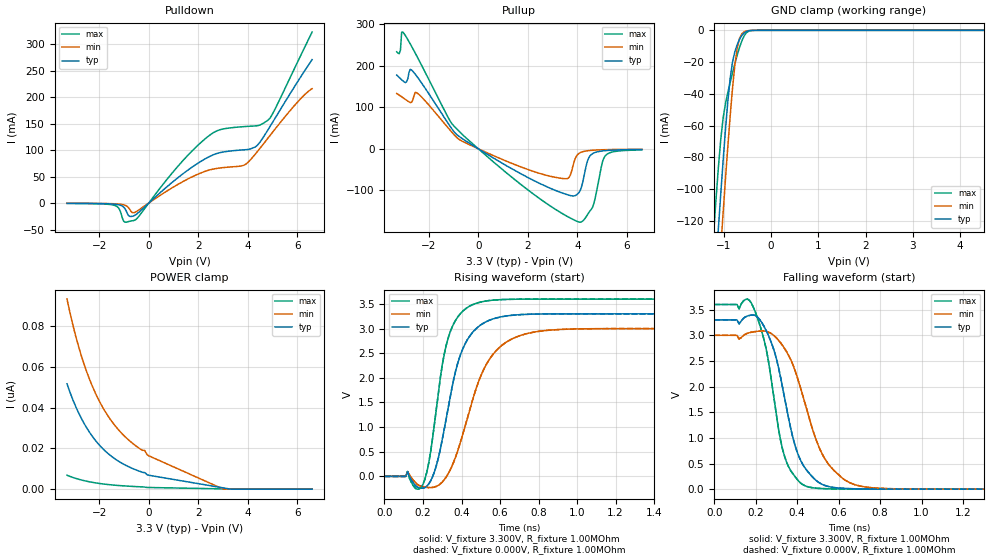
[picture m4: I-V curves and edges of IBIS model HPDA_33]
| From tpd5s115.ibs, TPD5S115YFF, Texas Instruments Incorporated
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[Model]   HPDA_33
Model_type   I/O
Vinl = 0.4V
Vinh = 1.0V
Vmeas = 1.500V
Vref = 0V
Cref =15pF
|   typ   min   max
|3-state
C_comp   1.7706pF   1.6054pF   2.0294pF
|pulldown
|C_comp   1.8194pF   1.5857pF   2.1620pF
|pullup
|C_comp   1.7863pF   1.5802pF   2.1259pF
[Voltage Range]   3.300V   3.000V   3.600V
|Junction temperature
[Temperature Range]   40.0   100.0   -40.0
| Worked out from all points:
|   slope of the pulldown table from 0 to 0.495 V, typ, clamps not added: 23.5 ohm
|   slope of the pullup table from 0 to 0.495 V, typ, clamps not added: 27.4 ohm
|   GND clamp passes 1 mA (typ) near -0.53 V on its own axis
|   falling waveform, V_fixture 3.300V, R_fixture 1.00MOhm: 20-80 % time 113ps typ, 151ps min, 91.6ps max; typ from 3.3 V to 0 V
|   rising waveform, V_fixture 3.300V, R_fixture 1.00MOhm: 20-80 % time 117ps typ, 162ps min, 89ps max; typ from 0 V to 3.3 V
|   rising waveform, V_fixture 0.000V, R_fixture 1.00MOhm: 20-80 % time 117ps typ, 162ps min, 89ps max; typ from 0 V to 3.3 V
|   falling waveform, V_fixture 0.000V, R_fixture 1.00MOhm: 20-80 % time 113ps typ, 151ps min, 91.6ps max; typ from 3.3 V to 0 V
|ambient temperature   25   85   -40
[Pulldown]
|   Voltage   I(typ)   I(min)   I(max)
-3.3V     -391uA     -285uA     -527uA
-1.41V    -1.95mA    -1.198mA   -3.883mA
-1.211V   -3.189mA   -1.754mA   -9.597mA
-961.8mV  -10.24mA   -3.813mA   -36.03mA
-762.8mV  -25.12mA   -12.16mA   -34.27mA
-514.1mV  -21.65mA   -16.26mA   -30.78mA
1.177V    47.93mA    35.3mA     69.48mA
2.371V    85.92mA    61.49mA    125mA
3.864V    100.7mA    72.03mA    144.6mA
4.361V    108.1mA    95.71mA    146.1mA
4.859V    141.5mA    125.2mA    158.4mA
6.6V      271mA      216.2mA    323.1mA
[GND Clamp]
|   Voltage   I(typ)   I(min)   I(max)
-3.3V     -1.186A    -1.22A     -1.144A
-1.211V   -169.5mA   -204.8mA   -127.5mA
-1.111V   -124.7mA   -159.3mA   -86.27mA
-1.061V   -103.1mA   -137mA     -68.77mA
-1.012V   -82.28mA   -115.2mA   -55.34mA
-912.1mV  -44.94mA   -73.37mA   -39.23mA
-812.6mV  -19.97mA   -36.53mA   -26.78mA
-713.1mV  -8.993mA   -11.15mA   -15.56mA
-663.3mV  -5.661mA   -5.005mA   -10.67mA
-563.8mV  -1.565mA   -864.6uA   -3.359mA
-364.8mV  -27.29uA   -19.88uA   -28.06uA
6.6V      0A         0A         0A
[Pullup]
|   Voltage   I(typ)   I(min)   I(max)
-3.3V     177.7mA    133.3mA    233.7mA
-3.151V   169.2mA    127.5mA    237.8mA
-3.051V   163.8mA    123.4mA    281.3mA
-2.703V   190mA      112.1mA    247.3mA
-2.454V   172mA      133.6mA    219.5mA
-1.061V   47.37mA    39.35mA    59.93mA
2.123V    -72.8mA    -52.26mA   -104.5mA
3.615V    -110.8mA   -70.96mA   -163.5mA
4.013V    -108.3mA   -13.48mA   -175.3mA
4.61V     -11.58mA   -3.356mA   -140.7mA
5.157V    -4.116mA   -1.942mA   -14.77mA
6.6V      -1.493mA   -912uA     -2.304mA
[POWER Clamp]
|   Voltage   I(typ)   I(min)   I(max)
-3.3V     51.61nA    93.19nA    6.828nA
-3.002V   42nA       77.47nA    5.491nA
-2.703V   34.29nA    64.67nA    4.449nA
-2.355V   27.23nA    52.76nA    3.519nA
-2.007V   21.8nA     43.44nA    2.82nA
-1.609V   17.12nA    35.23nA    2.228nA
-1.211V   13.63nA    28.98nA    1.791nA
-613.6mV  9.93nA     22.11nA    1.325nA
-165.8mV  8.144nA    19.03nA    1.055nA
-66.33mV  7.095nA    16.93nA    850.1pA
3.018V    614.7pA    0A         135.8pA
6.6V      0A         0A         0A
[Ramp]
R_load = 1.00MOhm
|   typ   min   max
dV/dt_r   1.980V/116.948ps   1.800V/161.908ps   2.160V/88.985ps
dV/dt_f   1.980V/113.008ps   1.800V/150.775ps   2.160V/91.589ps
[Falling Waveform]
V_fixture = 3.300V
V_fixture_min = 3.000V
V_fixture_max = 3.600V
R_fixture = 1.00MOhm
|   Time   V(typ)   V(min)   V(max)
0s        3.3V       3V         3.6V
180ps     3.395V     3.061V     3.621V
230ps     3.245V     3.085V     3.069V
270ps     2.915V     3.047V     2.283V
340ps     1.768V     2.739V     630.8mV
390ps     851.4mV    2.312V     243.2mV
440ps     402.2mV    1.644V     62.6mV
540ps     63.51mV    552.1mV    8.277mV
690ps     6.195mV    74.23mV    1.543mV
2ns       88.28uV    107.9uV    68.52uV
[Rising Waveform]
V_fixture = 3.300V
V_fixture_min = 3.000V
V_fixture_max = 3.600V
R_fixture = 1.00MOhm
|   Time   V(typ)   V(min)   V(max)
0s        88.28uV    107.9uV    68.52uV
120ps     92.2mV     88.43mV    99.35mV
200ps     -239.7mV   -209.5mV   -161.6mV
260ps     99.97mV    -216.8mV   1.076V
330ps     1.371V     46.89mV    2.798V
380ps     2.291V     513.4mV    3.233V
450ps     2.887V     1.446V     3.472V
560ps     3.192V     2.46V      3.577V
740ps     3.29V      2.899V     3.599V
2ns       3.3V       3V         3.6V
[Rising Waveform]
V_fixture = 0.000V
V_fixture_min = 0.000V
V_fixture_max = 0.000V
R_fixture = 1.00MOhm
|   Time   V(typ)   V(min)   V(max)
0s        12.66uV    15.32uV    11.71uV
120ps     92.12mV    88.34mV    99.3mV
200ps     -239.8mV   -209.7mV   -161.7mV
260ps     99.72mV    -217.1mV   1.076V
330ps     1.37V      46.55mV    2.798V
380ps     2.291V     513mV      3.233V
450ps     2.887V     1.446V     3.472V
560ps     3.192V     2.46V      3.577V
740ps     3.29V      2.899V     3.599V
2ns       3.3V       3V         3.6V
[Falling Waveform]
V_fixture = 0.000V
V_fixture_min = 0.000V
V_fixture_max = 0.000V
R_fixture = 1.00MOhm
|   Time   V(typ)   V(min)   V(max)
0s        3.3V       3V         3.6V
180ps     3.395V     3.061V     3.621V
230ps     3.245V     3.085V     3.069V
270ps     2.914V     3.046V     2.283V
340ps     1.768V     2.739V     630.7mV
390ps     851.2mV    2.311V     243.1mV
440ps     402.1mV    1.644V     62.54mV
540ps     63.42mV    552mV      8.22mV
690ps     6.119mV    74.11mV    1.486mV
2ns       12.66uV    15.32uV    11.71uV
